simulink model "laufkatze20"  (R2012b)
settings: Solver=ode45  StartTime=0.0  StopTime=50.0  RelTol=1e-3
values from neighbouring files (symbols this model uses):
  D = 0    [aktiv_tilger_1.m]    (also in aktiv_tilger_12.m; aktiv_tilger_3.m = 2000; aktiv_tilger_31.m; beobachter_1.m)
  g = 9.89    [fuellstnd_1.m]    (also in fuellstnd_2.m; fuellstnd_21.m; fuellstnd_3.m; fuellstnd_31.m)
  I = 2000    [aktiv_tilger_1.m]    (also in aktiv_tilger_12.m; aktiv_tilger_3.m = 0; aktiv_tilger_31.m = 0; fuellstnd_2.m = 0.0225)
  JL = 400    [laufkatze_1.m]    (also in laufkatze_10.m; laufkatze_2.m; laufkatze_20.m)
  ls = 4    [laufkatze_1.m]    (also in laufkatze_10.m; laufkatze_2.m; laufkatze_20.m)
  mk = 100    [laufkatze_1.m]    (also in laufkatze_10.m; laufkatze_2.m; laufkatze_20.m)
  mL = 500    [laufkatze_1.m]    (also in laufkatze_10.m; laufkatze_2.m; laufkatze_20.m)
  mu = 0.01    [laufkatze_10.m]    (also in laufkatze_20.m; feder_masse_1.m = 0.05; feder_masse_13.m = 0.05; feder_masse_14.m = 0.05)
  P = 0    [aktiv_tilger_1.m]    (also in aktiv_tilger_12.m; aktiv_tilger_3.m; aktiv_tilger_31.m; fuellstnd_2.m = 0.09)
  xsoll = 10    [laufkatze_2.m]    (also in laufkatze_20.m)
libraries: simulink x1

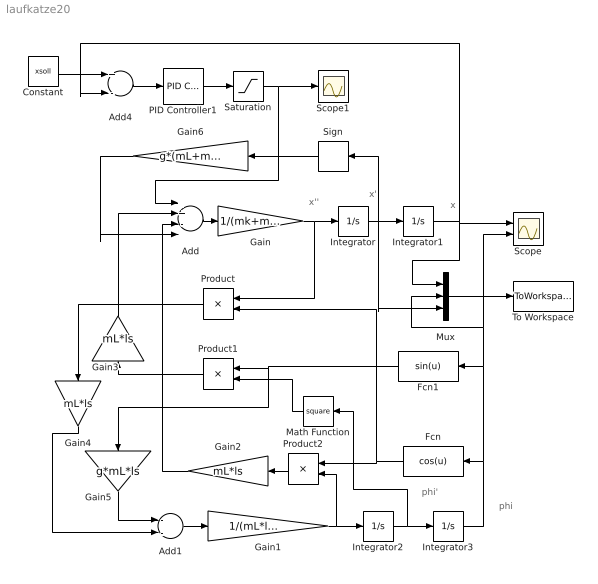
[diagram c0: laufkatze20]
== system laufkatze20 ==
  note: phi'
  note: x''
  note: x'
  note: x
  note: phi
  Add : Sum  Inputs=++--
  Add1 : Sum  Inputs=--
  Add4 : Sum  Inputs=+-
  Constant : Constant  Value=xsoll
  Fcn : Fcn  Expr=cos(u)
  Fcn1 : Fcn  Expr=sin(u)
  Gain : Gain  Gain=1/(mk+mL)
  Gain1 : Gain  Gain=1/(mL*ls*ls+JL)
  Gain2 : Gain  Gain=mL*ls
  Gain3 : Gain  Gain=mL*ls
  Gain4 : Gain  Gain=mL*ls
  Gain5 : Gain  Gain=g*mL*ls
  Gain6 : Gain  Gain=g*(mL+mk)*mu
  Integrator{,1..3} (4 alike) : Integrator
  Math Function : Math  Operator=square
  Mux : Mux  Inputs=3
  PID Controller1 : simulink/Continuous/PID Controller  Controller=PID  TimeDomain=Continuous-time  SampleTime=1  IntegratorMethod=Forward Euler  FilterMethod=Forward Euler  Form=Parallel  P=P  I=I  D=D  N=100  InitialConditionSource=internal  InitialConditionForIntegrator=0  InitialConditionForFilter=0  ExternalReset=none  LimitOutput=off  UpperSaturationLimit=inf  LowerSaturationLimit=-inf  LinearizeAsGain=on  AntiWindupMode=none  Kb=1  TrackingMode=off  Kt=1  PParamMin=[]  PParamMax=[]  IParamMin=[]  IParamMax=[]  DParamMin=[]  DParamMax=[]  NParamMin=[]  NParamMax=[]  KbParamMin=[]  KbParamMax=[]  KtParamMin=[]  KtParamMax=[]  POutMin=[]  POutMax=[]  IOutMin=[]  IOutMax=[]  DOutMin=[]  DOutMax=[]  NOutMin=[]  NOutMax=[]  KbOutMin=[]  KbOutMax=[]  KtOutMin=[]  KtOutMax=[]  IntegratorOutMin=[]  IntegratorOutMax=[]  FilterOutMin=[]  FilterOutMax=[]  SumOutMin=[]  SumOutMax=[]  SumI1OutMin=[]  SumI1OutMax=[]  SumI2OutMin=[]  SumI2OutMax=[]  SumI3OutMin=[]  SumI3OutMax=[]  SumDOutMin=[]  SumDOutMax=[]  SaturationOutMin=[]  SaturationOutMax=[]  IntegratorContinuousStateAttributes=''  IntegratorStateMustResolveToSignalObject=off  IntegratorRTWStateStorageClass=Auto  FilterContinuousStateAttributes=''  FilterStateMustResolveToSignalObject=off  FilterRTWStateStorageClass=Auto
  Product : Product
  Product1 : Product
  Product2 : Product
  Saturation : Saturate  UpperLimit=500  LowerLimit=-500
  Scope : Scope  NumInputPorts=2
  Scope1 : Scope
  Sign : Signum  ZeroCross=off
  To Workspace : ToWorkspace  VariableName=y  SampleTime=-1  SaveFormat=Structure With Time
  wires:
  Add/1 -> Gain/1
  Gain/1 -> Product/1, Integrator/1
  Integrator/1 -> Sign/1, Mux/3, Integrator1/1
  Add1/1 -> Gain1/1
  Gain1/1 -> Product2/2, Integrator2/1
  Integrator3/1 -> Fcn1/1, Scope/2, Mux/2, Fcn/1
  Fcn/1 -> Product/2, Product2/1
  Fcn1/1 -> Gain5/1, Product1/1
  Product2/1 -> Gain2/1
  Gain2/1 -> Add/3
  Math Function/1 -> Product1/2
  Integrator2/1 -> Math Function/1, Integrator3/1
  Product1/1 -> Gain3/1
  Gain3/1 -> Add/2
  Product/1 -> Gain4/1
  Gain5/1 -> Add1/1
  Integrator1/1 -> Add4/2, Scope/1, Mux/1
  Mux/1 -> To Workspace/1
  Constant/1 -> Add4/1
  Add4/1 -> PID Controller1/1
  PID Controller1/1 -> Saturation/1
  Saturation/1 -> Scope1/1, Add/1
  Gain4/1 -> Add1/2
  Sign/1 -> Gain6/1
  Gain6/1 -> Add/4
